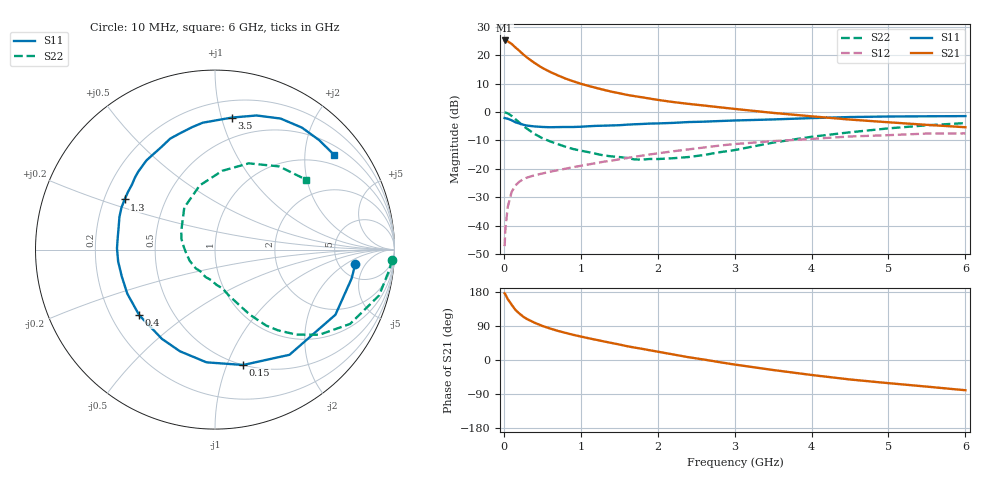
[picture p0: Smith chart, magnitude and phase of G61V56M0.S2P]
! SIEMENS Small Signal Semiconductors
! BFG193
! Si NPN RF Bipolar Junction Transistor in SOT223
! VCE = 1.5 V  IC = 6 mA
! Common Emitter S-Parameters:  August  1996
# GHz  S  MA  R  50
!  f  S11  S21  S12  S22
! GHz  MAG  ANG  MAG  ANG  MAG  ANG  MAG  ANG
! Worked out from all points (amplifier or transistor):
!   36 points, 10 MHz to 6 GHz, reference 50 ohm
!   highest |S21| = 25.2 dB at 10 MHz (marker M1)
!   |S21| within 3 dB of that: start of sweep to 174.2 MHz
!   unconditionally stable (mu >= 1): 1.009 GHz to 2.774 GHz
!   at 250 MHz: K = 0.39, MSG = 22.0 dB, |S12| = -23.6 dB
!   at 1.4 GHz: K = 1.09, MAG = 10.3 dB, |S12| = -17.1 dB
!   at 6 GHz: K = 0.94, MSG = 1.1 dB, |S12| = -7.5 dB
!   S11 on the Smith chart (normalised r, x): 10 MHz: 7.10, -2.96; 150 MHz: 0.50, -1.14; 400 MHz: 0.32, -0.34; 1.3 GHz: 0.29, +0.24; 3.5 GHz: 0.33, +1.08; 6 GHz: 0.72, +2.70
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0.01  0.7862 -5.8  18.09 176.0  0.0044 88.6  0.987 -3.3
0.02  0.7779 -12.0  18.08 173.1  0.0087 88.5  0.9794 -6.3
0.05  0.7628 -28.4  17.49 161.0  0.0212 75.3  0.9493 -15.6
0.1  0.7181 -54.7  15.78 146.4  0.0391 65.2  0.8593 -28.8
0.15  0.6616 -76.3  13.66 132.4  0.0512 55.4  0.7505 -39.2
0.2  0.6299 -94.3  11.96 122.9  0.0595 49.9  0.6565 -46.2
0.25  0.5993 -109.0  10.37 114.7  0.0659 45.4  0.5712 -52.0
0.3  0.5786 -120.7  9.109 108.2  0.0705 42.9  0.5108 -56.0
0.4  0.5584 -139.1  7.267 98.4  0.0775 39.8  0.4117 -61.8
0.5  0.5469 -153.3  5.96 89.9  0.0832 38.3  0.3475 -65.6
0.6  0.5405 -163.9  5.079 83.2  0.0894 38.0  0.3057 -69.0
0.7  0.5437 -173.0  4.415 77.0  0.095 38.0  0.2737 -72.5
0.9  0.5461 172.8  3.472 66.5  0.1076 38.1  0.2243 -78.4
1.1  0.5628 161.1  2.876 57.5  0.12 38.0  0.1973 -87.3
1.3  0.5758 151.0  2.453 49.0  0.1342 37.3  0.1727 -96.2
1.6  0.5999 138.0  2.003 36.5  0.1559 34.9  0.1557 -114.1
2.2  0.6448 117.6  1.498 14.7  0.2043 27.1  0.1543 -156.2
2.8  0.6943 100.5  1.214 -5.6  0.257 16.6  0.1963 162.4
3.5  0.7413 82.8  0.966 -26.4  0.3085 1.0  0.2903 126.1
4.5  0.8165 63.4  0.737 -51.4  0.3718 -18.7  0.441 84.7
5.5  0.8419 46.4  0.595 -70.3  0.4186 -42.7  0.5852 52.4
6  0.8481 38.4  0.541 -79.8  0.4221 -56.3  0.6394 37.6
